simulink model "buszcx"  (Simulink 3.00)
settings: Solver=VariableStepDiscrete  StartTime=0.0  StopTime=10  MaxStep=.05  RelTol=1e-3
libraries: simulink3 x2

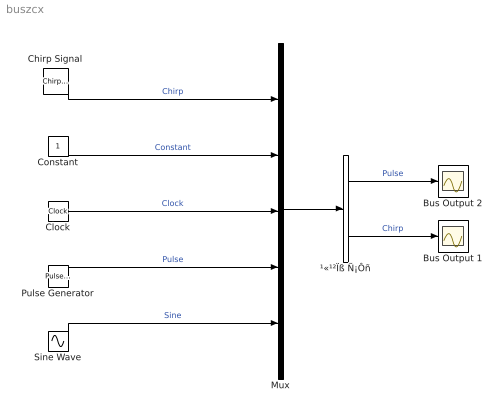
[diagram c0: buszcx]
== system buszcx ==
  Bus Output 1 : Scope
  Bus Output 2 : Scope
  Chirp Signal : simulink3/Sources/Chirp Signal  f1=0.1  T=10  f2=5
  Clock : Clock
  Constant : Constant  Value=1
  Mux : Mux  Inputs=5
  Pulse Generator : simulink3/Sources/Pulse Generator  period=1  duty=50  amplitude=1  start=0
  Sine Wave : Sin  Amplitude=1  Frequency=1  Phase=0  SampleTime=0
  ¹«¹²Ïß Ñ¡Ôñ : BusSelector  OutputSignals=Pulse,Chirp  MuxedOutput=off
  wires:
  Mux/1 -> ¹«¹²Ïß Ñ¡Ôñ/1
  Clock/1 -> Mux/3  "Clock"
  Pulse Generator/1 -> Mux/4  "Pulse"
  Sine Wave/1 -> Mux/5  "Sine"
  Chirp Signal/1 -> Mux/1  "Chirp"
  Constant/1 -> Mux/2  "Constant"
  ¹«¹²Ïß Ñ¡Ôñ/2 -> Bus Output 1/1  "Chirp"
  ¹«¹²Ïß Ñ¡Ôñ/1 -> Bus Output 2/1  "Pulse"
